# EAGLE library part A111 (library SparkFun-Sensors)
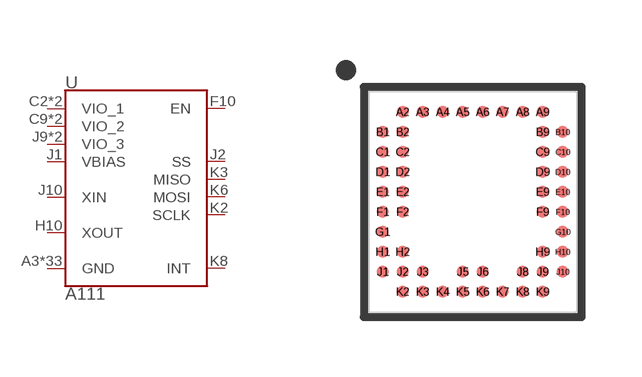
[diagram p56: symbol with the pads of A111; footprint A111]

Designator prefix U

## A111 (PROD_ID: IC-14498)  [A111]
A3  GND
A4  GND
A5  GND
A6  GND
A7  GND
A8  GND
A9  GND
B2  GND
B9  GND
B10  GND
C1  GND
C2  VIO_1
C9  VIO_2
C10  GND
D1  VIO_1
D2  GND
D9  GND
D10  VIO_2
E1  GND
E2  GND
E9  GND
E10  GND
F1  GND
F2  GND
F9  GND
F10  EN
G1  GND
G10  GND
H1  GND
H2  GND
H9  GND
H10  XOUT
J1  VBIAS
J2  SS
J3  GND
J5  GND
J6  GND
J8  GND
J9  VIO_3
J10  XIN
K2  SCLK
K3  MISO
K4  GND
K5  GND
K6  MOSI
K7  GND
K8  INT
K9  VIO_3

## Footprint A111 (pad centres in mm)
smd 0.3 x 0.3: A2 -1.75,2.25; A3 -1.25,2.25; A4 -0.75,2.25; A5 -0.25,2.25; A6 0.25,2.25; A7 0.75,2.25; A8 1.25,2.25; A9 1.75,2.25; B1 -2.25,1.75; B2 -1.75,1.75; B9 1.75,1.75; B10 2.25,1.75; C1 -2.25,1.25; C2 -1.75,1.25; C9 1.75,1.25; C10 2.25,1.25; D1 -2.25,0.75; D2 -1.75,0.75; D9 1.75,0.75; D10 2.25,0.75; E1 -2.25,0.25; E2 -1.75,0.25; E9 1.75,0.25; E10 2.25,0.25; F1 -2.25,-0.25; F2 -1.75,-0.25; F9 1.75,-0.25; F10 2.25,-0.25; G1 -2.25,-0.75; G10 2.25,-0.75; H1 -2.25,-1.25; H2 -1.75,-1.25; H9 1.75,-1.25; H10 2.25,-1.25; J1 -2.25,-1.75; J2 -1.75,-1.75; J3 -1.25,-1.75; J5 -0.25,-1.75; J6 0.25,-1.75; J8 1.25,-1.75; J9 1.75,-1.75; J10 2.25,-1.75; K2 -1.75,-2.25; K3 -1.25,-2.25; K4 -0.75,-2.25; K5 -0.25,-2.25; K6 0.25,-2.25; K7 0.75,-2.25; K8 1.25,-2.25; K9 1.75,-2.25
